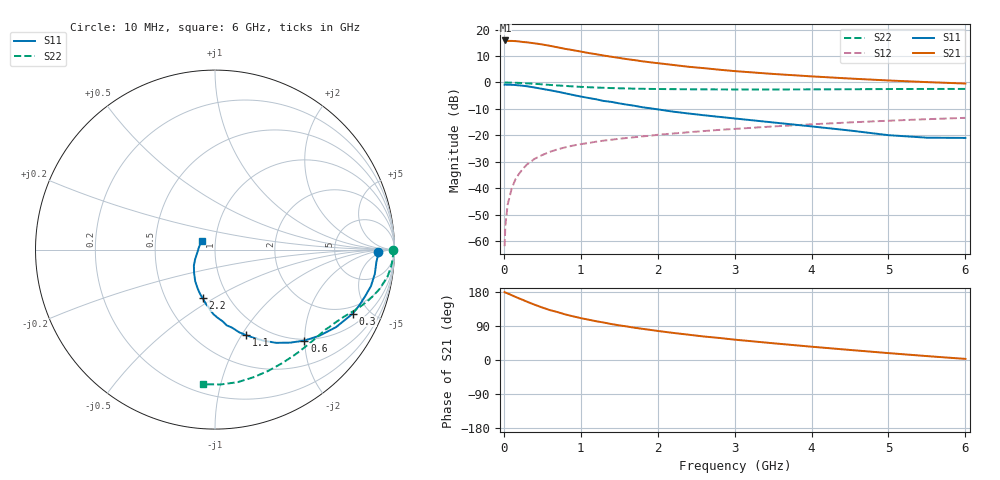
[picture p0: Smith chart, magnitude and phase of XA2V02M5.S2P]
! SIEMENS Discrete & RF Semiconductors
! BFY180
! Si NPN RF Bipolar Junction Transistor in MICRO-X
! VCE = 2 V  IC = 2.5 mA
! Common Emitter S-Parameters:  May  1997
# GHz  S  MA  R  50
!  f  S11  S21  S12  S22
! GHz  MAG  ANG  MAG  ANG  MAG  ANG  MAG  ANG
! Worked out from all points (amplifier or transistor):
!   36 points, 10 MHz to 6 GHz, reference 50 ohm
!   highest |S21| = 15.9 dB at 20 MHz (marker M1)
!   |S21| within 3 dB of that: start of sweep to 767.5 MHz
!   unconditionally stable (mu >= 1): 2.056 GHz to end of sweep
!   at 250 MHz: K = 0.17, MSG = 23.9 dB, |S12| = -32.6 dB
!   at 1.4 GHz: K = 0.83, MSG = 15.7 dB, |S12| = -21.7 dB
!   at 6 GHz: K = 1.10, MAG = 4.6 dB, |S12| = -13.4 dB
!   S11 on the Smith chart (normalised r, x): 10 MHz: 20, -3; 300 MHz: 1.57, -3.94; 600 MHz: 0.97, -1.99; 1.1 GHz: 0.82, -1.05; 2.2 GHz: 0.76, -0.45; 6 GHz: 0.86, +0.08
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0.01  0.9056 -0.9  6.083 179.2  0.0008 80.8  0.9935 -0.2
0.02  0.9093 -1.7  6.213 178.0  0.002 92.9  0.9942 -0.7
0.05  0.9018 -4.4  6.095 175.7  0.0049 83.1  0.9925 -1.8
0.1  0.9007 -8.6  6.095 171.2  0.0096 86.9  0.9897 -3.8
0.2  0.8769 -17.0  5.943 162.4  0.0189 80.3  0.9788 -7.3
0.3  0.8462 -24.9  5.732 153.9  0.028 74.8  0.9607 -10.6
0.4  0.8013 -32.6  5.48 145.9  0.0359 70.8  0.9415 -13.6
0.5  0.7542 -39.5  5.221 138.4  0.0424 66.6  0.9186 -16.3
0.6  0.7109 -45.5  4.911 131.6  0.0487 63.5  0.8964 -18.7
0.8  0.6216 -56.7  4.303 120.2  0.0593 58.7  0.8572 -22.7
1  0.5406 -65.9  3.829 110.5  0.0681 54.8  0.8237 -26.0
1.1  0.5083 -69.9  3.599 106.5  0.0715 53.6  0.8106 -27.4
1.2  0.4794 -73.8  3.412 102.3  0.0756 52.2  0.8 -28.9
1.5  0.4014 -84.0  2.902 91.4  0.0859 49.3  0.7738 -33.1
1.8  0.3391 -94.4  2.508 82.3  0.0953 47.5  0.7572 -37.1
2.2  0.2799 -104.3  2.139 71.5  0.108 44.7  0.7452 -42.5
2.6  0.2393 -113.5  1.86 62.0  0.1202 42.3  0.7387 -47.8
3  0.2081 -122.0  1.636 53.7  0.1321 39.5  0.7359 -53.0
3.5  0.1749 -131.8  1.446 44.2  0.1469 36.4  0.7349 -59.6
4.5  0.123 -154.1  1.183 26.5  0.1751 29.1  0.7428 -73.2
5.5  0.0901 170.8  1.013 10.3  0.2015 21.2  0.7521 -87.6
6  0.0891 147.3  0.952 2.9  0.2137 16.9  0.7531 -94.9
